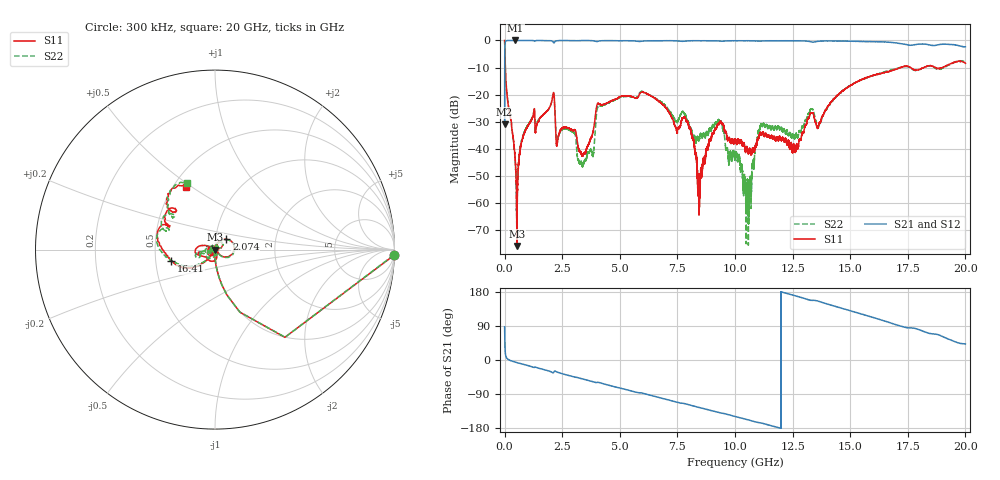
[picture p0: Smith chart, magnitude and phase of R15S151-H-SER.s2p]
!{R15S151}
!Johanson Technology Inc.
!www.johansontechnology.com
!Test Board Conditions:
!Substrate Type  RO4350B
!Substrate Thickness  20 mil
!Substrate Dk  3.66
!TL Type: GCPW
!TL Trace Width  34 mil
!TL Gap  10 mil
!Electrode orientation  Horizontal
!DUT TOPOLOGY	SERIES
!Mounting Pad LxW  26x52 mil
! Created Sat Feb  6 14:14:12 2021
# hz S ma R 50
! 2 Port Network Data from SP1.SP block
! freq  magS11  angS11  magS21  angS21  magS12  angS12  magS22  angS22
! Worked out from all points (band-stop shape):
!   20001 points, 300 kHz to 20 GHz, reference 50 ohm
!   highest |S21| = 0.00 dB at 467.3 MHz (marker M1); lowest = -31.0 dB at 300 kHz (marker M2)
!   |S21| within 3 dB of the highest: 10.75 MHz to end of sweep
!   lowest |S11| = -75.9 dB at 539.3 MHz (marker M3), VSWR 1.00, Z = 50 + j0.00128 ohm
!   |S11| at or under -10 dB: 31.86 MHz to 17.19 GHz (17.16 GHz wide, 199 % of centre); 17.62 GHz to 18.2 GHz (579.1 MHz wide, 3.23 % of centre); 18.71 GHz to 19 GHz (293.6 MHz wide, 1.56 % of centre)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
!   |S22| runs from -75.9 to 0.0 dB; largest |S21 - S12| = 0.017
!   S11 on the Smith chart (normalised r, x): 300 kHz: 5, -62; 2.074 GHz: 1.13, +0.13; 16.41 GHz: 0.60, -0.08; 20 GHz: 0.59, +0.47
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300000  0.9976 -1.8  0.02819 87.7  0.02823 88.1  0.9963 -1.7
1.063e8  0.09706 -85.7  0.9951 4.1  0.9945 4.1  0.09762 -85.8
4.673e8  0.005595 -95.9  1 -5.7  0.9989 -5.7  0.005341 -98.1
5.393e8  0.0001607 4.6  0.9998 -6.9  0.9994 -6.9  0.0007508 113.3
9.013e8  0.02155 78.1  0.9992 -12.9  0.999 -12.9  0.02224 77.5
2.0743e9  0.08569 42.2  0.9716 -33.0  0.9718 -33.0  0.08592 39.8
2.3043e9  0.01442 36.7  0.9923 -32.5  0.992 -32.5  0.01451 26.5
3.3343e9  0.008029 -19.7  0.9962 -49.2  0.9957 -49.1  0.005386 96.1
3.8193e9  0.01932 -80.8  0.9883 -57.3  0.989 -57.3  0.007593 -154.9
4.1123e9  0.06723 -125.9  0.9788 -59.7  0.9782 -59.6  0.06161 -144.7
6.6673e9  0.07709 162.1  0.987 -98.4  0.9878 -98.4  0.07909 -171.1
7.8903e9  0.03318 164.0  0.9799 -116.2  0.9807 -116.2  0.03679 -162.4
8.4603e9  0.001679 -155.9  0.9873 -125.6  0.9874 -125.5  0.01537 -108.3
9.3043e9  0.02846 -82.6  0.9749 -138.9  0.9767 -139.0  0.03355 -78.8
1.00003e10  0.01535 -118.5  0.9878 -148.9  0.9873 -148.9  0.007268 -53.4
1.05473e10  0.009684 -132.4  0.9867 -157.5  0.986 -157.6  0.002717 -44.9
1.11503e10  0.01882 147.5  0.9745 -166.5  0.9754 -166.5  0.02729 147.4
1.25633e10  0.01192 -11.7  0.986 170.4  0.9858 170.3  0.01664 165.1
1.33343e10  0.0457 -144.7  0.9368 157.4  0.9363 157.3  0.0542 -171.7
1.64093e10  0.2511 -165.5  0.941 104.6  0.9332 104.5  0.2589 -166.8
1.66673e10  0.2653 -172.3  0.93 99.4  0.9161 99.4  0.2786 -171.5
2e10  0.3794 114.4  0.7648 42.4  0.7576 42.3  0.4015 112.9
